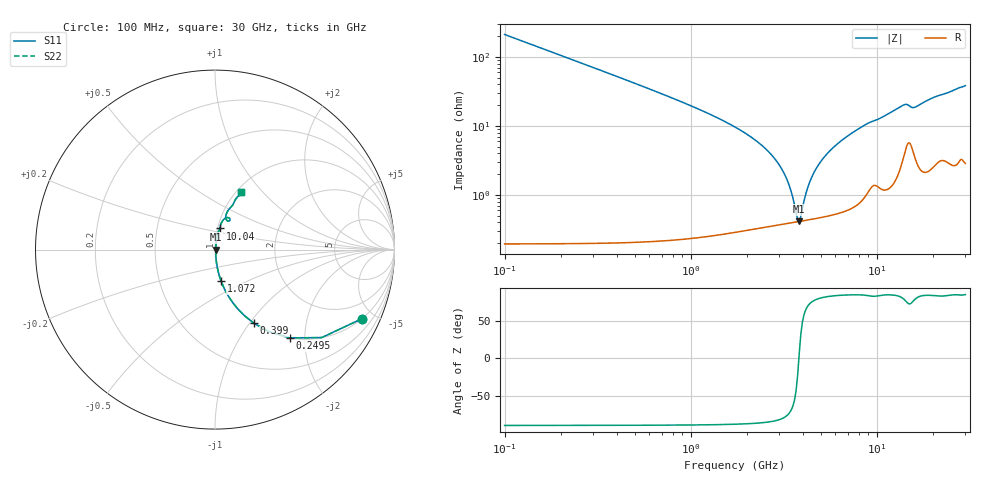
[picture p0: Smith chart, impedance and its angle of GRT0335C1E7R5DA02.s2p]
!Murata Part Number: GRT0335C1E7R5DA02
!These Parameters are Measured in Series Mode Connection
!Data Generated on Jun 19, 2026
!  o--ll--o
!Port1  Port2
!  o------o
!Operation Temp=25[degC], DC Bias Voltage=0[V]
!Freq. Start=100[MHz] Stop=30[GHz] 401[Steps]
# Hz S RI R 50
!Freq.(Hz) S11(Real) S11(Imag) S21(Real) S21(Imag) S12(Real) S12(Imag) S22(Real) S22(Imag)
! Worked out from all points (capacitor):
!   401 points, 100 MHz to 30 GHz, reference 50 ohm
!   read as one part in series: C = 7.5 pF near 249.5 MHz
!   lowest |Z| = 417 mohm at 3.837 GHz (marker M1)
!   series resonance near 3.82 GHz, so ESL is about 230 pH
!   S11 on the Smith chart (normalised r, x): 100 MHz: 1.00, -4.24; 249.5 MHz: 1.00, -1.69; 399 MHz: 1.00, -1.05; 1.072 GHz: 1.00, -0.36; 10.04 GHz: 1.03, +0.25; 30 GHz: 1.06, +0.77
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1e8  0.8178 -0.3855  0.1822 0.3855  0.1822 0.3855  0.8178 -0.3855
2.495e8  0.4178 -0.492  0.5822 0.492  0.5822 0.492  0.4178 -0.492
3.99e8  0.2175 -0.4106  0.7825 0.4106  0.7825 0.4106  0.2175 -0.4106
6.2325e8  0.1003 -0.2972  0.8997 0.2972  0.8997 0.2972  0.1003 -0.2972
1.07175e9  0.0342 -0.1752  0.9658 0.1752  0.9658 0.1752  0.0342 -0.1752
2.9405e9  0.00449 -0.0289  0.9955 0.0289  0.9955 0.0289  0.00449 -0.0289
3.31425e9  0.0041 -0.0155  0.9959 0.0155  0.9959 0.0155  0.0041 -0.0155
3.688e9  0.00406 -0.00382  0.9959 0.00382  0.9959 0.00382  0.00406 -0.00382
3.8375e9  0.00412 0.000513  0.9959 -0.000513  0.9959 -0.000513  0.00412 0.000513
3.91225e9  0.00417 0.00262  0.9958 -0.00262  0.9958 -0.00262  0.00417 0.00262
4.21125e9  0.00442 0.0107  0.9956 -0.0107  0.9956 -0.0107  0.00442 0.0107
4.4355e9  0.00468 0.0164  0.9953 -0.0164  0.9953 -0.0164  0.00468 0.0164
5.10825e9  0.00578 0.0322  0.9942 -0.0322  0.9942 -0.0322  0.00578 0.0322
5.9305e9  0.00767 0.0496  0.9923 -0.0496  0.9923 -0.0496  0.00767 0.0496
7.05175e9  0.0112 0.0715  0.9888 -0.0715  0.9888 -0.0715  0.0112 0.0715
1.004175e10  0.0275 0.1178  0.9725 -0.1178  0.9725 -0.1178  0.0275 0.1178
1.01165e10  0.0276 0.1188  0.9724 -0.1188  0.9724 -0.1188  0.0276 0.1188
1.37045e10  0.0622 0.1772  0.9378 -0.1772  0.9378 -0.1772  0.0622 0.1772
1.505e10  0.0819 0.1616  0.9181 -0.1616  0.9181 -0.1616  0.0819 0.1616
2.005825e10  0.0815 0.229  0.9185 -0.229  0.9185 -0.229  0.0815 0.229
2.50665e10  0.1107 0.2731  0.8893 -0.2731  0.8893 -0.2731  0.1107 0.2731
3e10  0.1466 0.3182  0.8534 -0.3182  0.8534 -0.3182  0.1466 0.3182
